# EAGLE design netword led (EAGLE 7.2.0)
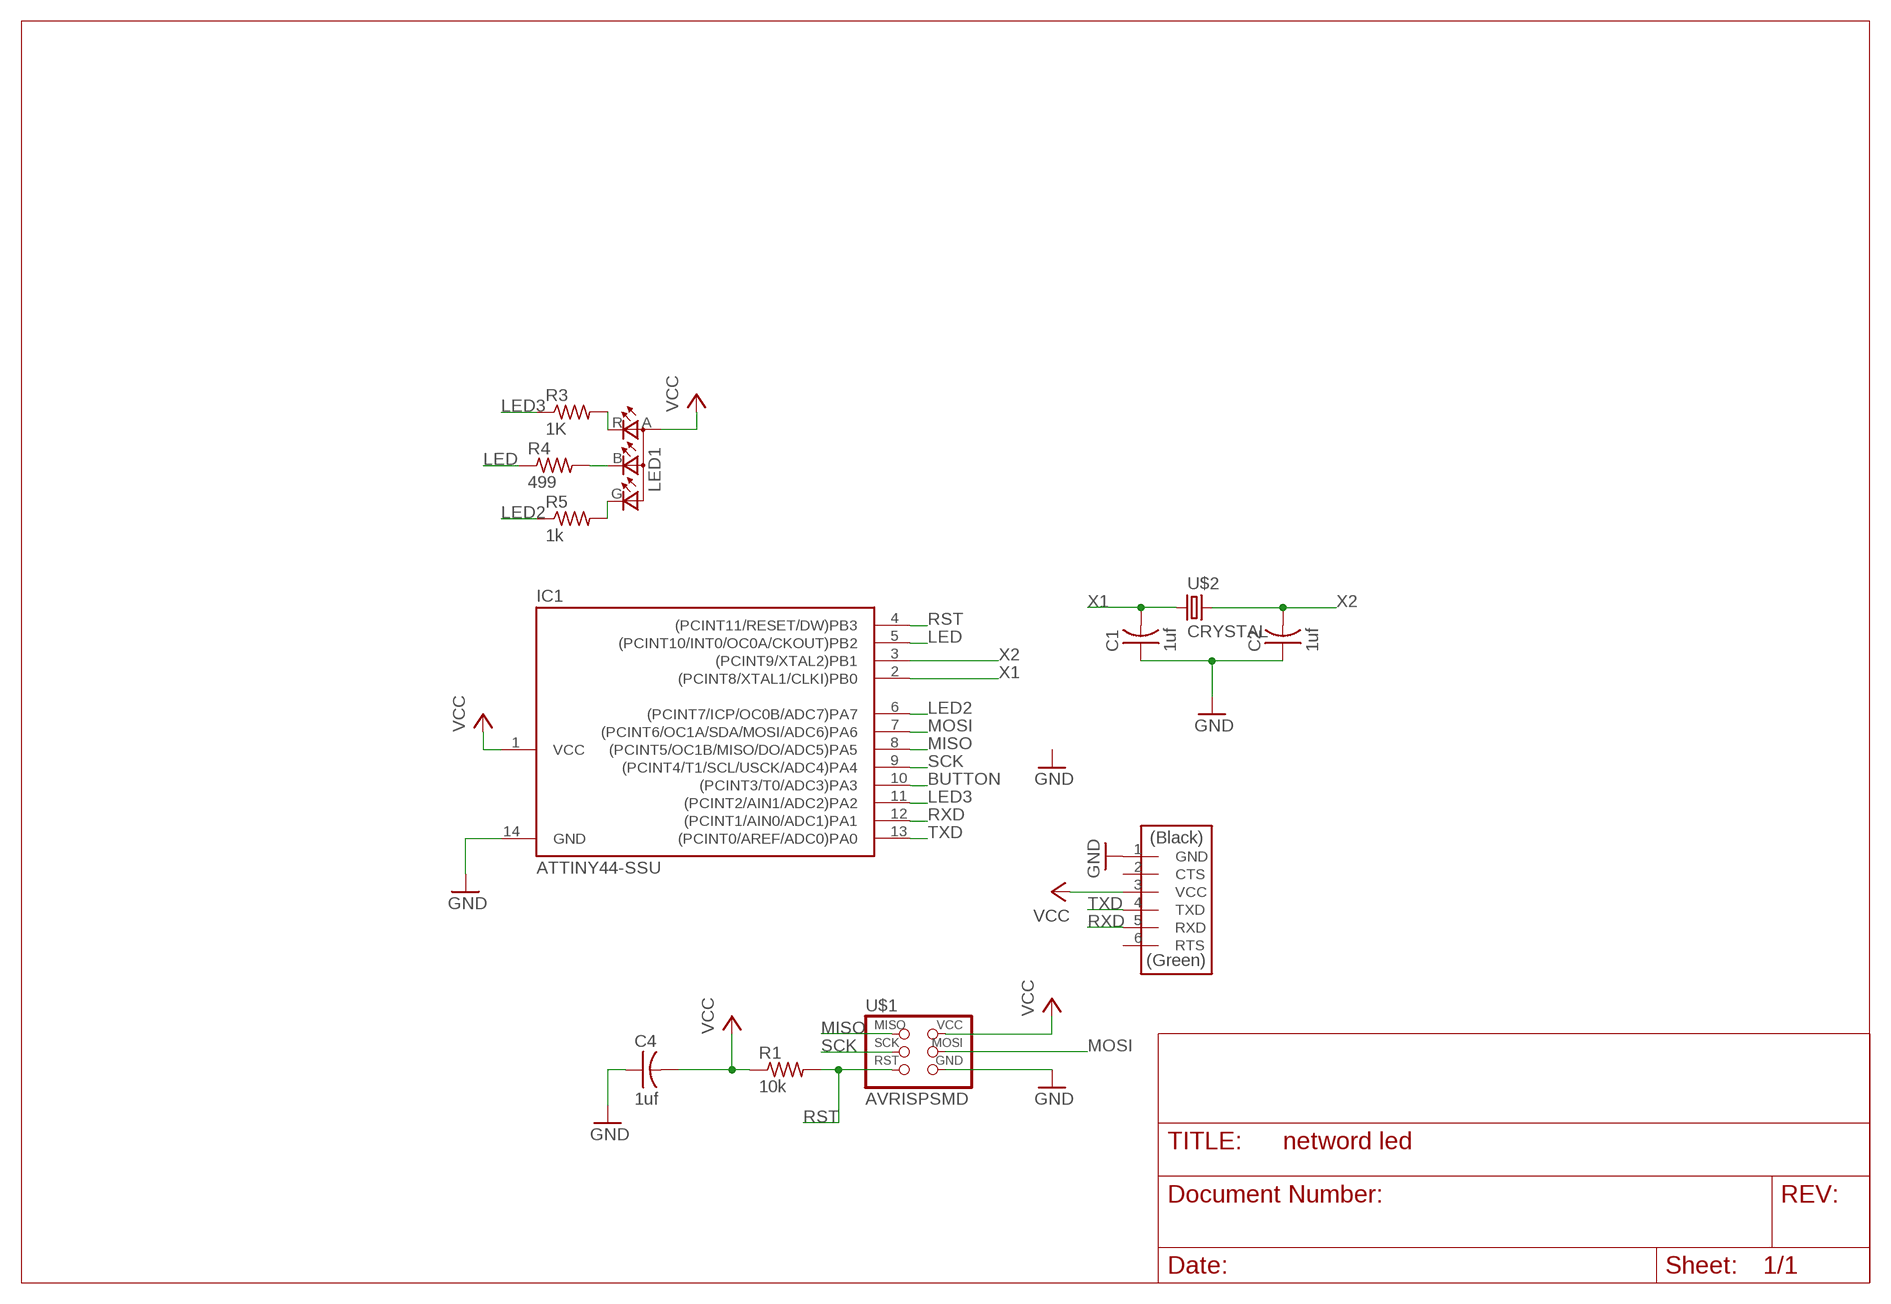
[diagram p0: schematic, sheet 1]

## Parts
C1  1uf  CAP-US1206FAB  [C1206FAB]
C2  1uf  CAP-US1206FAB  [C1206FAB]
C4  1uf  CAP-US1206FAB  [C1206FAB]
IC1  ATTINY44-SSU  [SOIC14]
LED1  LEDRGBOLD  [P-LCC-4-3]
R1  10k  RES-US1206FAB  [R1206FAB]
R3  1K  RES-US1206FAB  [R1206FAB]
R4  499  RES-US1206FAB  [R1206FAB]
R5  1k  RES-US1206FAB  [R1206FAB]
U$1  AVRISPSMD  [2X03SMD]
U$2  CRYSTAL  [2-SMD-5X3MM]
U$3  FTDI-SMD-HEADER  [1X06SMD]

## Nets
BUTTON: IC1.10((PCINT3/T0/ADC3)PA3)
GND: C1.1 C2.1 C4.1 IC1.14(GND) U$1.6(GND) U$3.1(GND)
LED: IC1.5((PCINT10/INT0/OC0A/CKOUT)PB2) R4.1
LED2: IC1.6((PCINT7/ICP/OC0B/ADC7)PA7) R5.1
LED3: IC1.11((PCINT2/AIN1/ADC2)PA2) R3.1
MISO: IC1.8((PCINT5/OC1B/MISO/DO/ADC5)PA5) U$1.1(MISO)
MOSI: IC1.7((PCINT6/OC1A/SDA/MOSI/ADC6)PA6) U$1.4(MOSI)
N$3: LED1.R(CRED) R3.2
N$4: LED1.B(CBLUE) R4.2
N$5: LED1.G(CGREEN) R5.2
RST: IC1.4((PCINT11/RESET/DW)PB3) R1.2 U$1.5(RST)
RXD: IC1.12((PCINT1/AIN0/ADC1)PA1) U$3.5(RXD)
SCK: IC1.9((PCINT4/T1/SCL/USCK/ADC4)PA4) U$1.3(SCK)
TXD: IC1.13((PCINT0/AREF/ADC0)PA0) U$3.4(TXD)
VCC: C4.2 IC1.1(VCC) LED1.A(A2) R1.1 U$1.2(VCC) U$3.3(VCC)
X1: C1.2 IC1.2((PCINT8/XTAL1/CLKI)PB0) U$2.P$1
X2: C2.2 IC1.3((PCINT9/XTAL2)PB1) U$2.P$2
Unconnected: U$3.2(CTS) U$3.6(RTS)

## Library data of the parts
C1 C2 C4 = fab:CAP-US
IC1 = fab:ATTINY44
LED1 = fab:LEDRGBOLD: OSRAM Hyper Multi TOPLED® Hyper-Bright LED LATB T686 Source: http://www.osram.convergy.de/
R1 R3-R5 = fab:RES-US: Resistor (US Symbol)
U$1 = fab:AVRISP
U$2 = 01fab:CRYSTAL
U$3 = fab:FTDI-SMD-HEADER

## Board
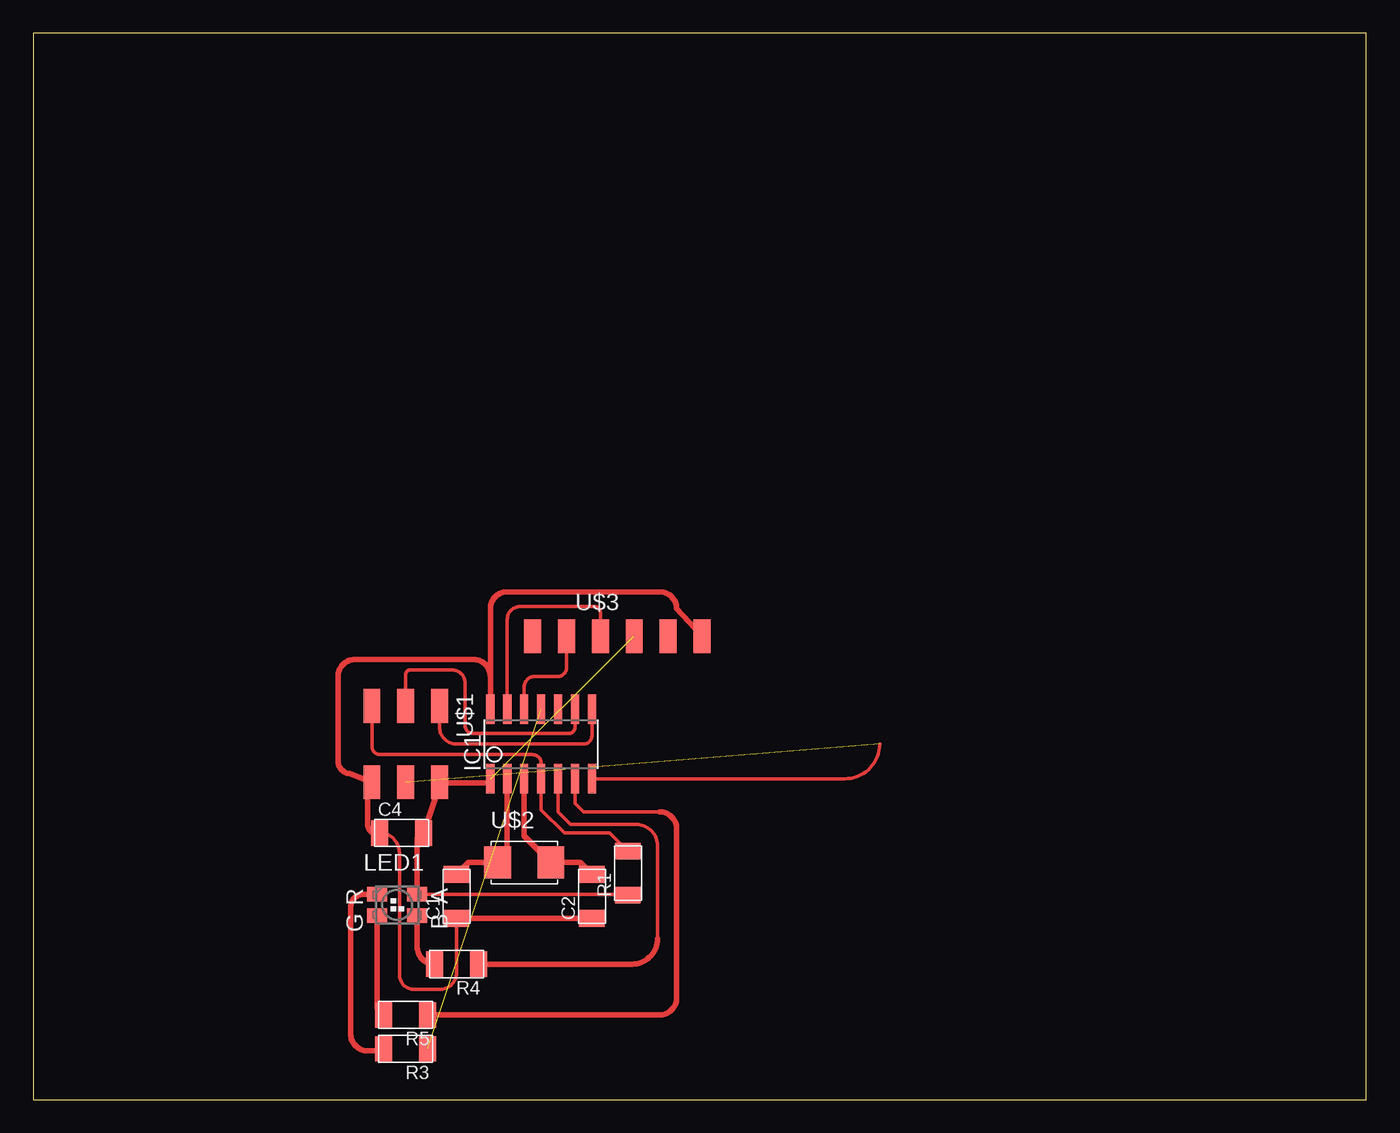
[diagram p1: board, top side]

Size 100 x 80 mm. Coordinates in mm from the lower left corner, seen from the top.
Outline: 0,0 100,0 100,80 0,80 0,0
Copper layers (1*16): Top 0.035mm / dielectric 1.5mm / Bottom 0.035mm
Design rules "default": minimum track width 10mil, minimum drill 24mil, track to track 8mil, track to pad 8mil, pad to pad 8mil, via to via 8mil, smd to smd 8mil, copper to edge 40mil, drill to drill 8mil, minimum pad ring 10mil, minimum via ring 8mil, stop-mask expansion 4mil, vias tented up to drill 0mil, thermal gap 10mil

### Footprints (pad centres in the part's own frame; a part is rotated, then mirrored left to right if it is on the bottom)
C1206FAB = smd 1.27 x 1.905: 1 -1.651,0; 2 1.651,0
SOIC14 = smd 0.61 x 2.21: 1 -3.81,-2.603; 2 -2.54,-2.603; 3 -1.27,-2.603; 4 0,-2.603; 5 1.27,-2.603; 6 2.54,-2.603; 7 3.81,-2.603; 8 3.81,2.603; 9 2.54,2.603; 10 1.27,2.603; 11 0,2.603; 12 -1.27,2.603; 13 -2.54,2.603; 14 -3.81,2.603
P-LCC-4-3 = smd 1.1 x 1.5: A -0.8,1.5; B 0.8,1.5; G 0.8,-1.5; R -0.8,-1.5
R1206FAB = smd 1.27 x 1.905: 1 -1.651,0; 2 1.651,0
2X03SMD = smd 2.54 x 1.27: 1 -2.857,2.54; 2 2.857,2.54; 3 -2.857,0; 4 2.857,0; 5 -2.857,-2.54; 6 2.857,-2.54
2-SMD-5X3MM = smd 2 x 2.4: P$1 -2,0; P$2 2,0
1X06SMD = smd 2.54 x 1.27: 1 0,6.35; 2 0,3.81; 3 0,1.27; 4 0,-1.27; 5 0,-3.81; 6 0,-6.35

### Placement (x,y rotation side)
C1  31.75,15.24 90 top
C2  41.91,15.24 90 top
C4  27.62,20 0 top
IC1  38.1,26.67 0 top
LED1  27.3,14.61 270 top
R1  44.61,16.99 90 top
R3  27.94,3.81 180 top
R4  31.75,10.16 180 top
R5  27.94,6.35 180 top
U$1  27.94,26.67 270 top
U$2  36.83,17.78 0 top
U$3  43.81,34.77 270 top

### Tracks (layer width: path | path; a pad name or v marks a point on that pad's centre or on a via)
GND
  Top 0.254: C4.1 arc-90 27.46,18.51 27.46,9.37 arc90 28.57,8.26 30.48,8.26 arc90 31.75,9.53 C1.1
  Top 0.406: C2.1 C1.1 | 34.29,31.75 arc90 33.02,33.02 24.13,33.02 arc90 22.86,31.75 22.86,25.4 arc90 23.81,24.45 U$1.6 25.4,23.18 | 34.29,31.75 IC1.14 | C4.1 25.72,20 arc-90 25.08,20.64 25.08,22.86 arc-90 25.4,23.18 | 25.4,23.18 25.4,22.86 | U$3.1 48.26,36.83 arc90 46.99,38.1 35.56,38.1 arc90 34.29,36.83 34.29,31.75
LED
  Top 0.254: 46.83,12.06 46.83,19.05 arc90 45.24,20.64 40.32,20.64 39.37,21.59 IC1.5
  Top 0.406: R4.1 44.93,10.16 arc90 46.83,12.06
LED2
  Top 0.254: 46.99,21.59 41.27,21.59 40.64,22.23 IC1.6
  Top 0.406: R5.1 46.99,6.35 arc90 48.26,7.62 48.26,20.32 arc90 46.99,21.59
LED3  (1 unrouted)
MISO
  Top 0.254: U$1.1 30.48,27.94 arc90 31.75,26.67 41.27,26.67 arc90 41.91,27.3 IC1.8
MOSI  (1 unrouted)
  Top 0.254: 41.91,24.13 IC1.7 60.9,24.07 arc90 63.5,26.67
N$3
  Top 0.406: LED1.R 24.77,15.4 arc90 23.81,14.45 23.81,4.92 arc90 25.08,3.65 26.13,3.65 arc90 R3.2
N$4
  Top 0.406: LED1.B 28.8,11.45 arc90 R4.2
N$5
  Top 0.406: LED1.G 25.8,6.83 arc90 R5.2
RST
  Top 0.254: U$1.5 25.4,26.51 arc90 26.04,25.88 37.47,25.88 arc-90 38.1,25.24 IC1.4 38.1,21.75 39.85,20 43.24,20 R1.2
RXD
  Top 0.254: U$3.5 40.01,32.38 arc-90 39.37,31.75 37.62,31.75 arc90 36.83,30.96 IC1.12
SCK
  Top 0.254: U$1.3 27.94,31.91 arc-90 28.26,32.23 31.43,32.23 arc-90 32.38,31.27 32.38,28.1 arc90 33.02,27.46 40.16,27.46 arc90 40.64,27.94 40.64,28.57 arc-90 40.8,28.73 40.8,29.11 arc90 IC1.9
TXD
  Top 0.254: IC1.13 35.56,36.04 arc-90 36.51,36.99 42.07,36.99 arc-90 42.55,36.51 U$3.4
VCC  (1 unrouted)
  Top 0.254: LED1.A 44.28,15.4 arc-90 44.45,15.24 44.51,15.24 arc90 R1.1
  Top 0.406: 30.54,23.75 C4.2 arc90 28.8,19.53 LED1.A | 30.54,23.75 arc90 U$1.2 | 30.54,23.75 33.97,23.75 arc90 IC1.1
X1
  Top 0.406: IC1.2 35.56,17.78 U$2.P$1 32.64,17.78 C1.2
X2
  Top 0.406: U$2.P$2 38.47,18.14 | 38.47,18.14 36.83,19.78 IC1.3 | C2.2 41.02,17.78 39.37,17.78 39.01,18.14 38.47,18.14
